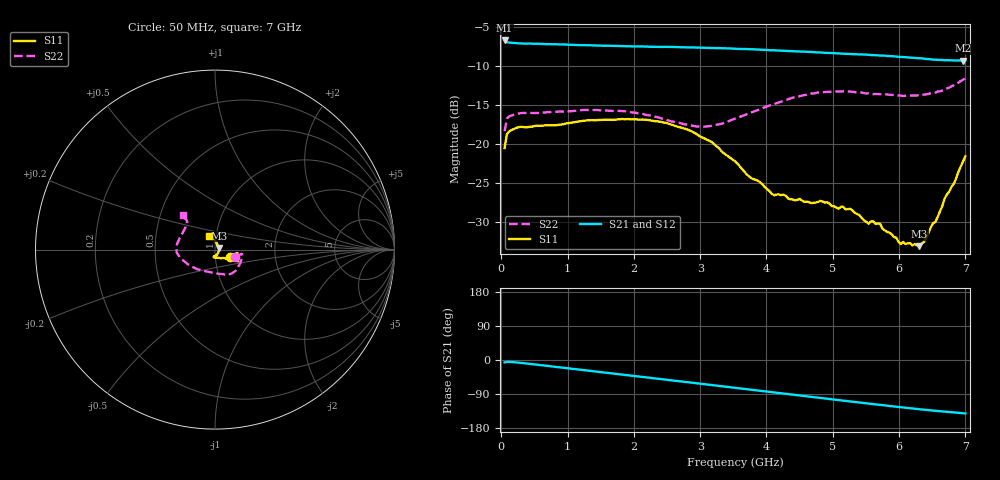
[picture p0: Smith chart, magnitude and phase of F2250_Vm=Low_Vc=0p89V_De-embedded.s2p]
! Integrated Device Technology
! Corporate Headquarters
! 6024 Silver Creek Valley Road
! San Jose, CA 95138  USA
! Phone:  1-408-284-8200
! Toll Free:  1-800-223-1366
! Webpage:  http://www.idt.com/
! Timing and RF Division
! 515 Groton Road, Suite 102
! Westford, MA 01886-6024
! Device:  F2250
! Description: Voltage Variable RF Attenuator
! Frequency:  50.0 -  6000.00 MHz
! Package:  3x3 mm Thin QFN Plastic Package: 16 pin
! Ports:  2 RF, 3 DC
!  Pin  1  = GND
!  Pin  2  = NC
!  Pin  3  = RF1  = Port 1
!  Pin  4  = NC
!  Pin  5  = GND
!  Pin  6  = GND
!  Pin  7  = GND
!  Pin  8  = GND
!  Pin  9  = NC
!  Pin 10  = RF2  = Port 2
!  Pin 11  = NC
!  Pin 12  = GND
!  Pin 13  = GND
!  Pin 14  = VCNTRL
!  Pin 15  = VDD
!  Pin 16  = VMODE
! Vcntrl:  0.890 Volts
! Vmode:  +0.000 Volts
! Vdd:  +3.30  Volts
! Current:  1.178 mA
! Data:  The device was measured on a the F2250 evaluation board which has
!  individual transmission lines to the RF pins.  Data was collected
!  using a calibrated network analyzer.  The evaluation board was
!  de-embedded using a TRL calibration technique.
!  The reference plane is the edge of the package pin.
! Misc:  SN 10
!  Action Tracker AT0258
! Date Measured:  2014-11-26
! Date:  2015-10-15  MJV
! Note:
!  Integrated Device Technology supplies this data as a sample of measured
!  data at the package pin for this product.  Your particular data for this
!  product may vary.
!  Data was taken at 25 degrees C.
!  Integrated Device Technology reserves the right to change this data at anytime.
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# GHz S dB R 50
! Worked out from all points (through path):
!   201 points, 50 MHz to 7 GHz, reference 50 ohm
!   highest |S21| = -6.76 dB at 50 MHz (marker M1); lowest = -9.4 dB at 6.965 GHz (marker M2)
!   group delay of S21, straight-line fit = 56.4 ps
!   lowest |S11| = -33.1 dB at 6.305 GHz (marker M3), VSWR 1.05, Z = 52.1 + j0.879 ohm
!   |S11| at or under -10 dB: start of sweep to end of sweep
!   |S22| runs from -18.4 to -11.6 dB; largest |S21 - S12| = 0.0013
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0.05  -20.56 -27.1  -6.76 -6.4  -6.76 -6.4  -18.40 -19.2
0.08475  -18.78 -13.5  -6.98 -5.2  -6.98 -5.1  -16.78 -10.8
0.22375  -17.99 -8.7  -7.12 -6.4  -7.12 -6.4  -16.22 -11.0
1.2315  -17.08 -23.9  -7.36 -26.6  -7.35 -26.6  -15.68 -42.4
2.37825  -17.16 -26.6  -7.59 -49.6  -7.59 -49.6  -16.65 -70.2
3.0385  -19.24 -29.7  -7.68 -63.4  -7.69 -63.4  -17.84 -101.4
3.525  -22.26 -40.4  -7.83 -73.6  -7.82 -73.6  -16.78 -130.3
4.11575  -26.62 -72.3  -8.02 -86.0  -8.01 -86.0  -14.92 -157.0
4.7065  -27.59 -99.3  -8.26 -98.2  -8.27 -98.2  -13.57 -173.4
4.81075  -27.34 -100.1  -8.30 -100.3  -8.31 -100.3  -13.40 -175.5
5.08875  -28.35 -98.9  -8.41 -106.0  -8.42 -106.0  -13.32 177.9
5.2625  -28.35 -91.8  -8.50 -109.4  -8.51 -109.4  -13.33 174.0
5.5405  -30.27 -79.5  -8.61 -115.0  -8.62 -115.0  -13.54 167.1
5.71425  -30.29 -64.8  -8.70 -118.5  -8.70 -118.5  -13.66 162.6
5.85325  -31.42 -53.3  -8.76 -121.2  -8.76 -121.2  -13.73 159.0
6.027  -32.87 -32.9  -8.88 -124.6  -8.87 -124.6  -13.83 153.6
6.305  -33.15 22.5  -9.05 -129.9  -9.03 -130.0  -13.76 144.3
6.54825  -30.05 67.3  -9.23 -134.1  -9.22 -134.1  -13.46 137.3
6.68725  -27.01 84.3  -9.30 -136.2  -9.29 -136.2  -13.01 134.4
6.82625  -25.14 99.3  -9.33 -138.2  -9.33 -138.3  -12.51 133.9
6.96525  -22.28 112.3  -9.36 -140.5  -9.35 -140.5  -11.79 133.7
7  -21.61 114.4  -9.33 -141.0  -9.33 -141.1  -11.60 133.3
